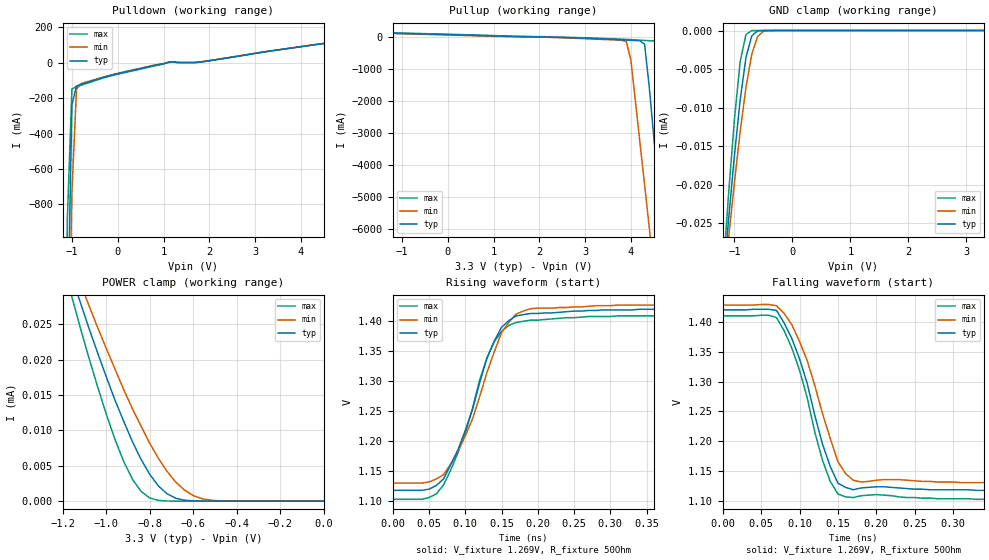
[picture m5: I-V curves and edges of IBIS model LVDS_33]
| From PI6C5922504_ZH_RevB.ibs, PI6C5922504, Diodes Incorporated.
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| Model  OUTPUT LVDS_33
[Model]  LVDS_33
Model_type  Output
Vmeas = 1.269
Rref = 50
|Variable   typ   min   max
C_comp   1.93p   1.91p  1.96p
|Variable   typ   min   max
[Voltage Range]   3.3   3.0   3.6
[Temperature Range]   25   85   -40
[Pullup Reference]   3.3   3.0   3.6
[Pulldown Reference]   0   0   0
[Power Clamp Reference]   3.3   3.0   3.6
[GND Clamp Reference]   0   0   0
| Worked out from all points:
|   slope of the pulldown table from 0 to 0.495 V, typ, clamps not added: 17.2 ohm
|   slope of the pullup table from 0 to 0.495 V, typ, clamps not added: 24.2 ohm
|   falling waveform, V_fixture 1.269V, R_fixture 50Ohm: 20-80 % time 40.8ps typ, 44.4ps min, 39ps max; typ from 1.42 V to 1.12 V
|   rising waveform, V_fixture 1.269V, R_fixture 50Ohm: 20-80 % time 50.4ps typ, 53.5ps min, 49.3ps max; typ from 1.12 V to 1.42 V
[gnd clamp]
-3.3V     -239uA     -209uA     -287uA
-1.2V     -33.2uA    -34.4uA    -31.9uA
-1.1V     -24.5uA    -26.9uA    -21.2uA
-1V       -16.3uA    -19.8uA    -11.6uA
-900mV    -9uA       -13.1uA    -4.02uA
-800mV    -3.48uA    -7.37uA    -510nA
-700mV    -692nA     -3.07uA    -12.5nA
-600mV    -51nA      -785nA     -109pA
-500mV    -1.49nA    -102nA     -9.86pA
-400mV    -38.9pA    -6.45nA    -8.8pA
3.3V      6.6pA      207pA      6pA
[power clamp]
-3.28V    253uA      224uA      299uA
-1.16V    31.8uA     34.1uA     29.1uA
-1.12V    28.2uA     30.9uA     24.6uA
-1.08V    24.5uA     27.7uA     20.3uA
-1V       17.6uA     21.6uA     12.3uA
-920mV    11.3uA     15.8uA     5.62uA
-840mV    5.91uA     10.6uA     1.38uA
-800mV    3.79uA     8.18uA     451nA
-760mV    2.14uA     6.04uA     105nA
-680mV    406nA      2.68uA     3.06nA
-560mV    8.78nA     347nA      19.3pA
0V        6.6pA      6.02pA     7.2pA
[Pulldown]
| Voltage   I(typ)   I(min)  I(max)
-3.3V     -36A       -30.7A     -44.9A
-1.2V     -3.12A     -3.33A     -2.88A
-1.1V     -1.55A     -2.03A     -879mA
-1V       -238mA     -727mA     -148mA
-900mV    -131mA     -149mA     -134mA
-800mV    -121mA     -118mA     -127mA
-200mV    -74.6mA    -72.5mA    -77.6mA
900mV     -10.2mA    -8.21mA    -13.3mA
1.1V      2.03mA     1.33mA     3.01mA
1.8V      4.2mA      4.89mA     3.56mA
3.3V      65.1mA     64.8mA     65.4mA
6.6V      188mA      188mA      189mA
[Pullup]   |Note: Vtable = Vcc - Voutput
| Voltage   I(typ)   I(min)  I(max)
-3.3V     188mA      176mA      200mA
2.2V      -14.4mA    -19.7mA    -4.36mA
3.9V      -106mA     -148mA     -86.6mA
4V        -113mA     -725mA     -93.2mA
4.2V      -129mA     -3.33A     -110mA
4.3V      -236mA     -4.63A     -118mA
4.4V      -1.55A     -5.94A     -126mA
4.6V      -4.68A     -8.54A     -147mA
4.7V      -6.24A     -9.85A     -879mA
4.9V      -9.37A     -12.5A     -4.88A
5V        -10.9A     -13.8A     -6.87A
6.6V      -36A       -34.6A     -38.9A
[Falling Waveform]
V_fixture = 1.269V
V_fixture_min = 1.279V
V_fixture_max = 1.256V
R_fixture = 50Ohm
C_fixture = 0F
|   Time   V(typ)   V(min)   V(max)
0s        1.42V      1.428V     1.41V
70ps      1.419V     1.427V     1.407V
100ps     1.338V     1.367V     1.319V
110ps     1.297V     1.335V     1.273V
130ps     1.195V     1.246V     1.168V
140ps     1.158V     1.205V     1.133V
150ps     1.13V      1.166V     1.112V
160ps     1.123V     1.146V     1.107V
180ps     1.122V     1.132V     1.109V
980ps     1.118V     1.13V      1.103V
[Rising Waveform]
V_fixture = 1.269V
V_fixture_min = 1.279V
V_fixture_max = 1.256V
R_fixture = 50Ohm
C_fixture = 0F
|   Time   V(typ)   V(min)   V(max)
0s        1.118V     1.13V      1.103V
50ps      1.12V      1.132V     1.106V
70ps      1.137V     1.144V     1.127V
90ps      1.186V     1.183V     1.181V
110ps     1.253V     1.237V     1.255V
130ps     1.339V     1.315V     1.339V
150ps     1.39V      1.381V     1.383V
170ps     1.409V     1.412V     1.398V
310ps     1.419V     1.427V     1.409V
970ps     1.42V      1.428V     1.41V
[Ramp]
|   typ   min   max
dV/dt_r   0.181/50.18E-12   0.1783/53.04E-12   0.1836/48.75E-12
dV/dt_f   0.181/41.11E-12   0.1783/44.27E-12   0.1836/39.38E-12
R_load =   50.0000
